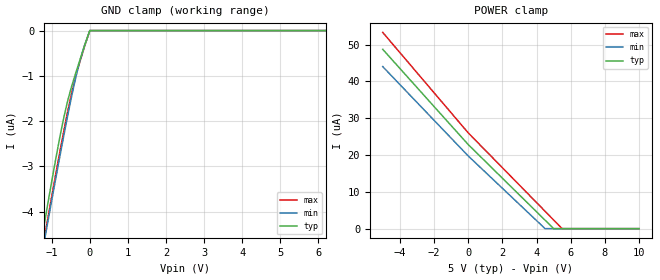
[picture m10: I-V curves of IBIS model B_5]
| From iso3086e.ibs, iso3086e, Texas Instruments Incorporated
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|   B_5 Model
[Model]   B_5
Model_type   Input
|Signals   B   negative pin
|Rref = 27   Note: 54 Ohm differential load;
Vinl   = 0.8
Vinh   = 2
| C_comp   obtained at 20MHz
|   typ   min   max
C_comp   5.334fF   5.274f   5.390fF
[Voltage Range]   5   4.5   5.5
[Temperature Range]   40   125   -40
[Power Clamp Reference]   5   4.5   5.5
[GND Clamp Reference]   0   0   0
[GND Clamp]
|   Voltage   I(typ)   I(min)   I(max)
-5V       -24.05uA   -23.38uA   -24.97uA
-1.295V   -4.787uA   -5.146uA   -5.082uA
-1.183V   -4.23uA    -4.617uA   -4.539uA
-1.16V    -4.119uA   -4.512uA   -4.431uA
-1.145V   -4.046uA   -4.442uA   -4.36uA
-792.5mV  -2.391uA   -2.821uA   -2.714uA
-605mV    -1.645uA   -1.995uA   -1.896uA
-440mV    -1.136uA   -1.317uA   -1.255uA
-290mV    -734.3nA   -776.7nA   -780.4nA
-140mV    -341.8nA   -335.3nA   -361.7nA
2.5mV     0A         0A         0A
10V       0A         0A         0A
[POWER Clamp]
|   Voltage   I(typ)   I(min)   I(max)
-5V       48.71uA    44.02uA    53.3uA
2.5mV     22.84uA    19.75uA    26.02uA
4.503V    2.294uA    0A         4.721uA
5.005V    0A         0A         2.343uA
5.5V      0A         0A         0A
10V       0A         0A         0A
